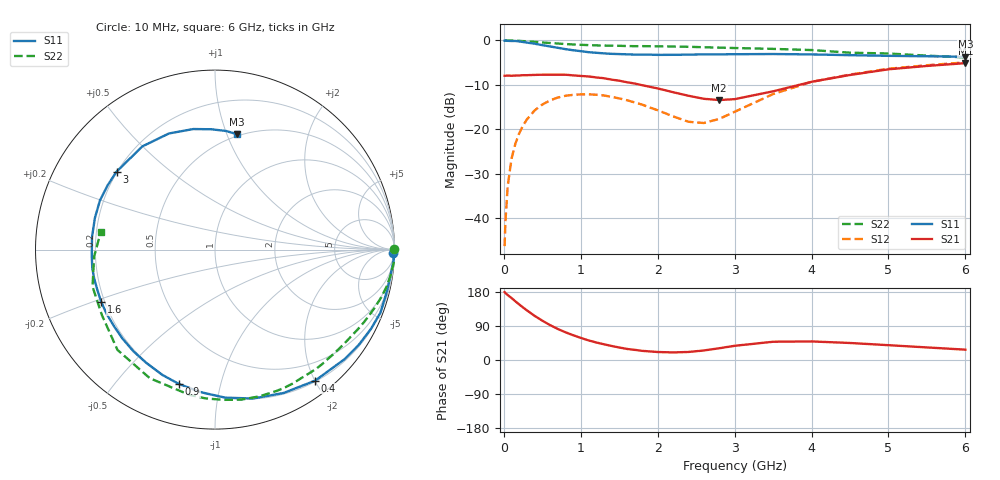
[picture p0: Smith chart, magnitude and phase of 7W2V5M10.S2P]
! Infineon Technologies  Discrete & RF Semiconductors
! BFS17W
! Si NPN RF Bipolar Junction Transistor in SOT323
! VCE = 2.5 V  IC = 0.1 mA
! Common Emitter S-Parameters:  August  1999
# GHz  S  MA  R  50
!  f  S11  S21  S12  S22
! GHz  MAG  ANG  MAG  ANG  MAG  ANG  MAG  ANG
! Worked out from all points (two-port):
!   36 points, 10 MHz to 6 GHz, reference 50 ohm
!   highest |S21| = -5.11 dB at 6 GHz (marker M1); lowest = -13.4 dB at 2.8 GHz (marker M2)
!   |S21| within 3 dB of the highest: start of sweep to 1.101 GHz; 4.393 GHz to end of sweep
!   lowest |S11| = -3.7 dB at 6 GHz (marker M3), VSWR 4.78, Z = 24.2 + j54.4 ohm
!   |S11| at or under -10 dB: nowhere
!   |S22| runs from -3.8 to 0.0 dB; largest |S21 - S12| = 0.4
!   S11 on the Smith chart (normalised r, x): 10 MHz: 25, -88; 400 MHz: 0.21, -2.01; 900 MHz: 0.20, -0.75; 1.6 GHz: 0.19, -0.21; 3 GHz: 0.20, +0.34; 6 GHz: 0.48, +1.09
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0.01  0.9941 -1.2  0.4 179.1  0.0048 90.1  0.9999 0.1
0.02  0.9971 -3.0  0.4 176.8  0.0089 92.8  0.9991 -0.9
0.05  0.99 -6.8  0.402 171.5  0.0227 85.8  0.9988 -2.1
0.1  0.9862 -13.3  0.4 163.5  0.0465 81.5  0.9987 -4.2
0.2  0.9746 -27.0  0.403 146.6  0.0899 72.7  0.9891 -8.3
0.3  0.9459 -40.1  0.406 131.0  0.1289 63.9  0.9781 -12.2
0.4  0.919 -52.6  0.409 116.5  0.1628 55.9  0.9636 -16.0
0.6  0.8561 -75.7  0.411 92.2  0.211 41.9  0.9355 -22.7
0.9  0.7756 -104.9  0.404 65.4  0.2438 25.5  0.901 -32.0
1.1  0.7378 -121.4  0.393 51.8  0.247 17.2  0.8862 -38.0
1.3  0.7152 -136.1  0.375 41.5  0.2398 10.4  0.8752 -44.3
1.6  0.6977 -155.4  0.338 29.2  0.2121 3.3  0.8651 -53.5
2.2  0.6888 174.2  0.261 20.0  0.1395 7.5  0.8541 -73.2
2.6  0.6972 156.8  0.22 25.1  0.1173 33.0  0.8384 -87.0
2.8  0.6972 149.1  0.213 31.0  0.1305 47.2  0.8304 -93.8
3  0.6996 141.6  0.218 37.4  0.157 56.8  0.8215 -100.1
3.5  0.7032 125.1  0.267 48.2  0.2487 62.8  0.8034 -116.9
4  0.696 111.6  0.342 49.0  0.3414 57.6  0.7795 -134.2
4.5  0.6825 100.2  0.408 44.9  0.4131 50.1  0.728 -150.0
5  0.6708 91.8  0.473 39.1  0.48 42.7  0.7128 -163.2
5.5  0.6637 84.6  0.516 33.2  0.5256 35.6  0.6743 -176.8
6  0.6541 79.1  0.555 27.3  0.5662 29.1  0.6442 171.4
